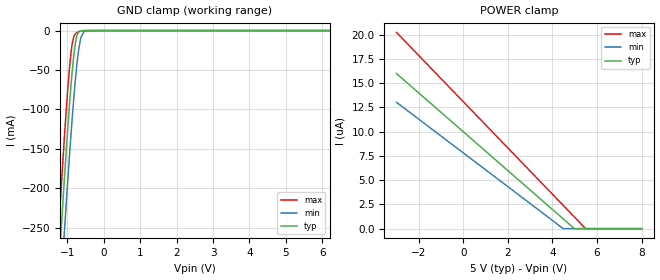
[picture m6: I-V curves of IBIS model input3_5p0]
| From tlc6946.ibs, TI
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|   input3_5p0 Model
[Model]   input3_5p0
Model_type   Input
Vinl = 1.5
Vinh = 3.5
|   typ   min   max
C_comp   1.3666pF   1.3478pF   1.3856pF
|  Where Nom  PVT is Nominal Process, 5.0V,   27C
|   Fast PVT is Strong Process,  5.5V,   -40C
|   Slow PVT is Weak Process,   4.5V,   105C
[Model spec]
|subparameter
Vinl   1.5   1.35   1.65
Vinh   3.5   3.15   3.85
[Voltage Range]   5   4.5   5.5
|Junction Temperature
[Temperature Range]   27   105   -40
[Power Clamp Reference]   5   4.5   5.5
[GND Clamp Reference]   0   0   0
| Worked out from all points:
|   GND clamp passes 1 mA (typ) near -0.66 V on its own axis
[GND Clamp]
|   Voltage   I(typ)   I(min)   I(max)
-3V       -1.709A    -1.711A    -1.711A
-1.251V   -312.6mA   -378.3mA   -260.9mA
-1.185V   -262.6mA   -329mA     -210.1mA
-1.086V   -189.9mA   -256.8mA   -137.3mA
-976mV    -114.6mA   -180.1mA   -65.34mA
-899mV    -67.8mA    -129.8mA   -27.03mA
-778mV    -15.07mA   -60.6mA    -4.072mA
-690mV    -1.835mA   -23.96mA   -1.294mA
-624mV    -337uA     -7.804mA   -375.2uA
-536mV    -37.71uA   -841.3uA   -42.56uA
-239mV    -453nA     -523.2nA   -542.6nA
8V        0A         0A         0A
[POWER Clamp]
|   Voltage   I(typ)   I(min)   I(max)
-3V       15.99uA    13.03uA    20.22uA
4.48V     1.017uA    8.272nA    2.407uA
4.986V    2.848nA    0A         1.202uA
5.481V    0A         0A         21.2nA
8V        0A         0A         0A
